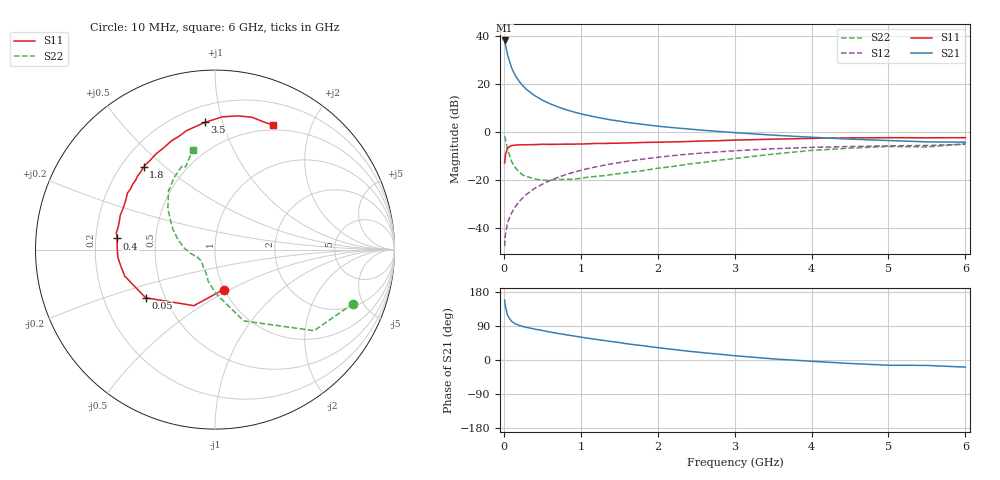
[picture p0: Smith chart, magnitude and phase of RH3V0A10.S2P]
! SIEMENS Small Signal Semiconductors
! BFR106
! Si NPN RF Bipolar Junction Transistor in SOT23
! VCE = 3 V  IC = 100 mA
! Common Emitter S-Parameters:  August  1996
# GHz  S  MA  R  50
!  f  S11  S21  S12  S22
! GHz  MAG  ANG  MAG  ANG  MAG  ANG  MAG  ANG
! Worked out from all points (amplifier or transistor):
!   36 points, 10 MHz to 6 GHz, reference 50 ohm
!   highest |S21| = 38.2 dB at 10 MHz (marker M1)
!   |S21| within 3 dB of that: start of sweep to 29.86 MHz
!   unconditionally stable (mu >= 1): 142.1 MHz to 2.855 GHz; 5.107 GHz to end of sweep
!   at 250 MHz: K = 1.09, MAG = 21.4 dB, |S12| = -27.3 dB
!   at 1.4 GHz: K = 1.08, MAG = 7.4 dB, |S12| = -13.2 dB
!   at 6 GHz: K = 1.01, MAG = -0.1 dB, |S12| = -5.1 dB
!   S11 on the Smith chart (normalised r, x): 10 MHz: 0.99, -0.47; 50 MHz: 0.39, -0.27; 400 MHz: 0.29, +0.05; 1.8 GHz: 0.29, +0.42; 3.5 GHz: 0.31, +0.88; 6 GHz: 0.44, +1.48
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0.01  0.2279 -78.0  81.11 158.2  0.0042 74.9  0.8269 -21.3
0.02  0.3337 -110.6  68.62 141.9  0.0072 70.0  0.7132 -39.3
0.05  0.4704 -145.2  39.91 116.8  0.0133 60.2  0.428 -68.1
0.1  0.5242 -163.6  22.02 102.1  0.0206 66.1  0.2447 -88.9
0.15  0.5353 -171.5  14.99 95.4  0.0279 69.3  0.1815 -101.9
0.2  0.5427 -175.4  11.38 91.4  0.0358 72.1  0.1465 -108.6
0.25  0.5435 -179.2  9.109 88.2  0.0433 72.8  0.1264 -117.5
0.3  0.5458 178.0  7.623 85.9  0.0514 73.4  0.1183 -122.8
0.4  0.5478 173.5  5.773 81.7  0.0671 74.0  0.1056 -132.5
0.5  0.5576 170.3  4.638 77.7  0.0822 73.6  0.0994 -139.2
0.6  0.554 166.2  3.891 73.9  0.098 72.5  0.0994 -143.4
0.7  0.5567 162.8  3.363 70.2  0.1136 71.6  0.1022 -147.6
0.9  0.5609 156.6  2.653 63.6  0.1447 68.7  0.104 -155.5
1.1  0.5704 150.2  2.212 57.3  0.1748 65.7  0.1155 -160.4
1.4  0.5854 141.7  1.786 48.8  0.2181 60.9  0.1303 -168.5
1.8  0.6082 130.9  1.454 38.0  0.2722 54.3  0.1562 -179.1
2.2  0.6263 121.6  1.236 27.9  0.3237 47.7  0.1921 170.1
2.8  0.6628 107.5  1.03 15.3  0.3887 37.7  0.2604 154.3
3.5  0.7111 94.5  0.864 3.0  0.4503 26.7  0.3481 139.0
4.5  0.756 80.1  0.714 -9.1  0.5001 12.2  0.4622 119.5
5.5  0.7614 68.7  0.625 -14.3  0.5263 3.1  0.4892 109.6
6  0.7658 64.9  0.616 -18.8  0.5572 -3.7  0.5702 102.5
